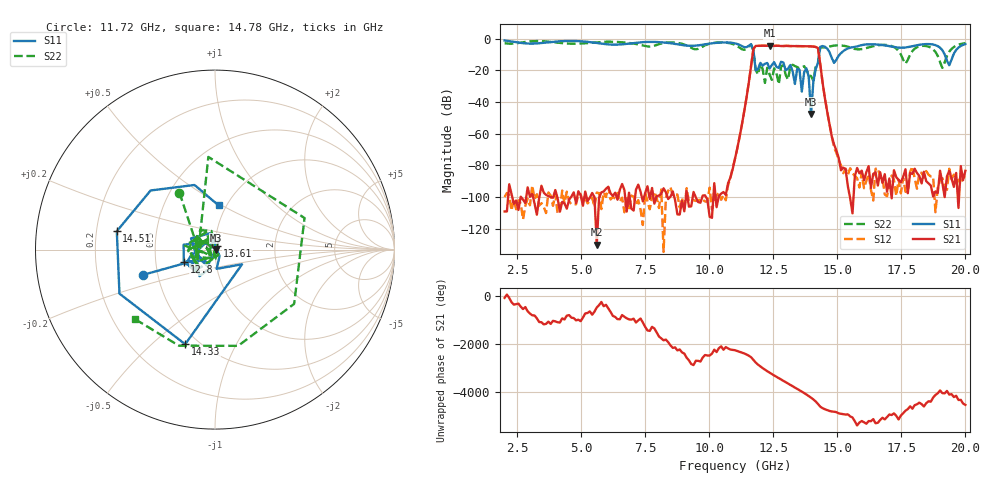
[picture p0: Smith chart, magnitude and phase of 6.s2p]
!Keysight Technologies,N5234A,MY52241180,A.10.60.03
!Date: Friday, January 20, 2023 09:34:22
!Correction: S11(Full 2 Port(1,2))
!S21(Full 2 Port(1,2))
!S12(Full 2 Port(1,2))
!S22(Full 2 Port(1,2))
!S2P File: Measurements: S11, S21, S12, S22:
# Hz S  dB  R 50
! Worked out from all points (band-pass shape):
!   201 points, 2 GHz to 20 GHz, reference 50 ohm
!   highest |S21| = -4.41 dB at 12.35 GHz (marker M1); lowest = -130.1 dB at 5.6 GHz (marker M2)
!   |S21| within 3 dB of the highest: 11.71 GHz to 14.25 GHz (2.543 GHz wide, 19.6 % of centre)
!   lowest |S11| = -47.6 dB at 13.97 GHz (marker M3), VSWR 1.01, Z = 50.4 - j0.208 ohm
!   |S11| at or under -10 dB: 11.74 GHz to 14.29 GHz (2.549 GHz wide, 19.6 % of centre); 14.73 GHz to 15.09 GHz (364 MHz wide, 2.44 % of centre); 19.19 GHz to 19.54 GHz (343.2 MHz wide, 1.77 % of centre)
!   |S22| runs from -28.8 to -1.5 dB; largest |S21 - S12| = 0.00073
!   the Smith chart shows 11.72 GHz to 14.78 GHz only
!   S11 on the Smith chart (normalised r, x): 11.72 GHz: 0.42, -0.14; 12.8 GHz: 0.70, -0.10; 13.61 GHz: 1.02, +0.04; 14.33 GHz: 0.42, -0.64; 14.51 GHz: 0.29, +0.09; 14.78 GHz: 0.92, +0.48
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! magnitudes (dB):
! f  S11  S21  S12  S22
! 2 GHz  -1.1  -109.2  -100.0  -2.8
! 5.06 GHz  -1.7  -105.6  -103.0  -3.0
! 5.6 GHz  -2.7  -130.1  -97.2  -2.3
! 8.03 GHz  -2.2  -99.1  -107.0  -3.5
! 11 GHz  -3.0  -75.7  -76.0  -4.0
! 11.72 GHz  -7.5  -6.4  -6.4  -8.5
! 11.81 GHz  -20.1  -4.6  -4.6  -19.8
! 12.35 GHz  -18.9  -4.4  -4.4  -22.6
! 12.8 GHz  -14.6  -4.6  -4.6  -17.6
! 13.52 GHz  -19.6  -4.7  -4.7  -18.8
! 13.61 GHz  -33.4  -4.7  -4.7  -18.3
! 13.79 GHz  -18.8  -4.8  -4.8  -19.5
! 13.97 GHz  -47.6  -4.9  -4.9  -23.6
! 14.06 GHz  -27.3  -5.0  -5.0  -26.6
! 14.33 GHz  -5.1  -16.0  -16.0  -5.7
! 14.51 GHz  -5.1  -37.4  -37.3  -5.4
! 14.78 GHz  -12.2  -61.8  -61.3  -4.6
! 15.14 GHz  -9.1  -83.2  -80.1  -4.3
! 17.03 GHz  -4.7  -88.3  -92.3  -4.2
! 19.1 GHz  -7.3  -91.2  -88.1  -18.5
! 19.37 GHz  -16.8  -83.5  -82.2  -8.2
! 20 GHz  -3.4  -83.5  -87.7  -2.8
